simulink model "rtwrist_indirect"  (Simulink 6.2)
settings: Solver=ode45  SolverMode=SingleTasking  StartTime=0.0  StopTime=inf  FixedStep=h  RelTol=1e-3  AbsTol=1e-6
PreLoadFcn:
  | hwinit
StartFcn:
  | hwinit
StopFcn:
  | rtunload
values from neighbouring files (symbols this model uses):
  adingain = [1.2*(pi*2/620/3)*[1 -1 -1 1 1 1] 1]    [hwinit.m]
  adinoffs = [-421 -511 -568 -518 -521 -410    0]    [hwinit.m]
  daoutgain = 127*[1 -1 -1 1 1 1 1]    [hwinit.m]
  daoutoffs = 127*[1 1 1 1 0.98 1 0]    [hwinit.m]
  h = 0.01    [design_pol.m]    (also in design_rot.m; design_wrist.m; rtrobot_init.m = 0.05; simpleregret.m = cfg.h)
  joint = [1 2 3 4 5]    [design_pol.m]    (also in design_rot.m = [1 5]; design_wrist.m = [5]; rtrobot_init.m = joint(:)+(0:6:6*(n-1))')
  Kd = [0.4 0.1 0.1]    [design_pol.m]    (also in design_rot.m = [0.3 0.1]; design_wrist.m = 0.01; mc_approx_vectorized.m = cfg.Kd)
  Ki = [0.6 0.3 0.9]/3    [design_pol.m]    (also in design_rot.m = [0.1 0.1]; design_wrist.m = 0)
  Kp = [0.5 0.2 1.0]    [design_pol.m]    (also in design_rot.m = [0.4 2]; design_wrist.m = 1.5)
undefined symbols (not defined in the file or in its folder): COM1, No
libraries: xpclib x4, rtlib x1, simulink x1

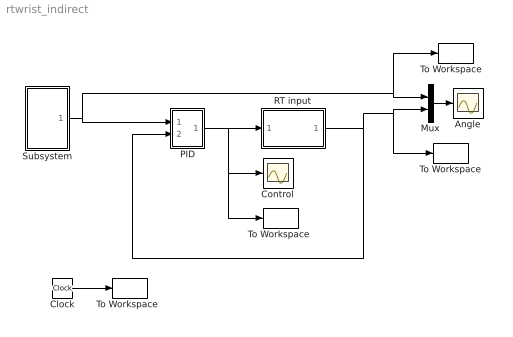
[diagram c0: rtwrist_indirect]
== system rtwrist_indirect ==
  Angle : Scope
  Clock : Clock
  Control : Scope
  Mux : Mux  Inputs=2
  PID : Subsystem
  RT input : Subsystem  InitFcn=rtclear all  mask{h=h, joint=joint, Port=COM1, laser=No, gripper=No}
      mask prompts: h "Sample time [s]:"; joint "Joints to control (e.g., [1 2 4])"; Port "Serial port:"; laser "Enable laser input"; gripper "Enable gripper current sensor"
      mask init:
      | hwinit;
      | sen = joint(:);                             % read joint angles
      | if strcmp(gripper,'Yes'),                   % if gripper current desired
      |     sen = [sen; 7];                         % add to the list
      | end;    
      |                                             
      | n = length(sen);                            % number of sensors to be read
      | sen = sen+(0:7:7*(n-1))';                   % convert into sequential index
      | sen_select = zeros(7,n);                    % prepare zeros
      | sen_select(sen) = 1;                        % assign 1 at the right places
      | 
      | act = joint(:);                             % control joint actuators
      | if strcmp(laser,'Yes'),                     % if laser desired
      |     act = [act; 7];                         % add to the list
      | end;    
      |                                             
      | n = length(act);                            % number of actuators to be controlled
      | act = act+(0:7:7*(n-1))';                   % convert into sequential index
      | act_select = zeros(7,n);                    % prepare zeros
      | act_select(act) = 1;                        % assign 1 at the right places
      | 
      | rtrobot_init(Port);
  Subsystem : Subsystem
  To Workspace : ToWorkspace  VariableName=y  SampleTime=h  SaveFormat=Array
  "To Workspace " : ToWorkspace  VariableName=u  SampleTime=h  SaveFormat=Array
  "To Workspace  " : ToWorkspace  VariableName=t  SampleTime=h  SaveFormat=Array
  "To Workspace   " : ToWorkspace  VariableName=r  SampleTime=h  SaveFormat=Array
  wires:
  Mux/1 -> Angle/1
  Subsystem/1(out_1) -> PID/1(in_1), Mux/1, "To Workspace   "/1
  RT input/1(Angles) -> PID/2(in_2), Mux/2, To Workspace/1
  PID/1(out_1) -> Control/1, "To Workspace "/1, RT input/1(Motors)
  Clock/1 -> "To Workspace  "/1

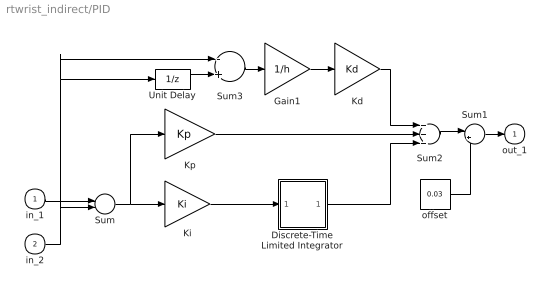
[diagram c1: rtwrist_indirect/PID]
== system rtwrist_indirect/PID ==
  in_1 : Inport  Port=1  LatchInput=off
  in_2 : Inport  Port=2  LatchInput=off
  Discrete-Time Limited Integrator : Subsystem  mask(Discrete-Time Limited Integrator.){}
      mask help: Discrete-Time Limited Integrator.
      mask init:
      | lower_limit=@1;upper_limit=@2;X0=@3;Ts=@4;
  Gain1 : Gain  Gain=1/h  SampleTime=h
  Kd : Gain  Gain=Kd  SampleTime=h
  Ki : Gain  Gain=Ki  SampleTime=h
  Kp : Gain  Gain=Kp  SampleTime=h
  Sum : Sum  Inputs=+-  SampleTime=h
  Sum1 : Sum  Inputs=|++
  Sum2 : Sum  Inputs=+++
  Sum3 : Sum  Inputs=-+  SampleTime=h
  Unit Delay : UnitDelay  SampleTime=h
  offset : Constant  Value=0.03
  out_1 : Outport  InitialOutput=0
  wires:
  Discrete-Time Limited Integrator/1(out_1) -> Sum2/3
  Ki/1 -> Discrete-Time Limited Integrator/1(in_1)
  Sum/1 -> Ki/1, Kp/1
  Gain1/1 -> Kd/1
  Sum3/1 -> Gain1/1
  Kp/1 -> Sum2/2
  Kd/1 -> Sum2/1
  Unit Delay/1 -> Sum3/2
  in_1/1 -> Sum/1
  in_2/1 -> Sum/2, Unit Delay/1, Sum3/1
  Sum2/1 -> Sum1/1
  Sum1/1 -> out_1/1
  offset/1 -> Sum1/2

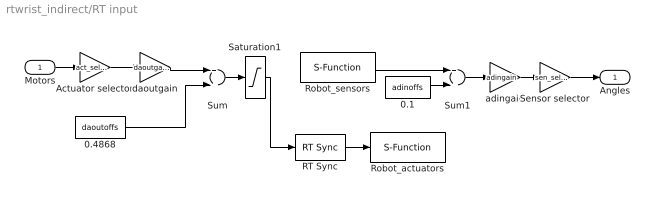
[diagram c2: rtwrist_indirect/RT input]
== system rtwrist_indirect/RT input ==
  Motors : Inport  Port=1  LatchInput=off
  0.1 : Constant  Value=adinoffs
  0.4868 : Constant  Value=daoutoffs
  Actuator selector : Gain  Gain=act_select  Multiplication=Matrix(K*u)
  RT Sync : rtlib/RT Sync
  Robot_actuators : S-Function  FunctionName=sfserialout  Parameters=Ts, com  mask(Serial Out){Ts=h, Port=Port}
      mask prompts: Ts "Sample time:"; Port "Serial port:"
      mask help: Serial line output block
      mask init:
      | com = xserial('Port',Port,'Baudrate',115200);
  Robot_sensors : S-Function  FunctionName=sfserialin  Parameters=Ts, com  mask(Serial Out){Ts=h, Port=Port}
      mask prompts: Ts "Sample time:"; Port "Serial port:"
      mask help: Serial line output block
      mask init:
      | com = xserial('Port',Port,'Baudrate',115200);
  Saturation1 : Saturate  UpperLimit=255  LowerLimit=0
  Sensor selector : Gain  Gain=sen_select'  Multiplication=Matrix(K*u)
  Sum : Sum
  Sum1 : Sum
  adingain : Gain  Gain=adingain
  daoutgain : Gain  Gain=daoutgain
  Angles : Outport
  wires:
  RT Sync/1 -> Robot_actuators/1
  Actuator selector/1 -> daoutgain/1
  Sensor selector/1 -> Angles/1
  Saturation1/1 -> RT Sync/1
  daoutgain/1 -> Sum/1
  adingain/1 -> Sensor selector/1
  Robot_sensors/1 -> Sum1/1
  0.1/1 -> Sum1/2
  Sum1/1 -> adingain/1
  Motors/1 -> Actuator selector/1
  0.4868/1 -> Sum/2
  Sum/1 -> Saturation1/1

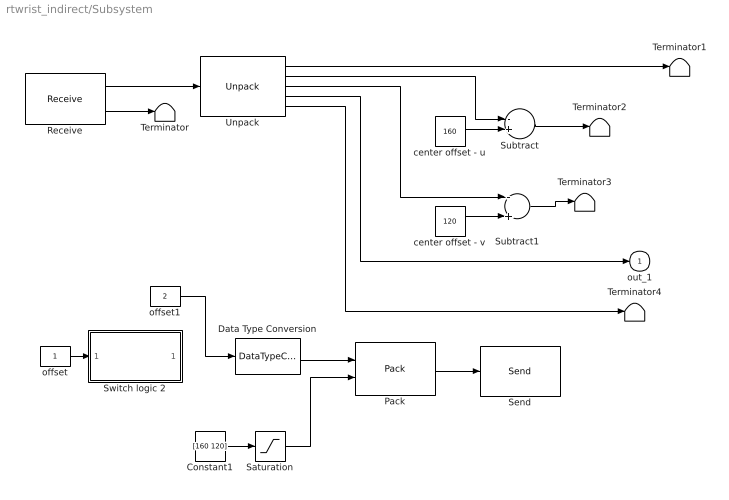
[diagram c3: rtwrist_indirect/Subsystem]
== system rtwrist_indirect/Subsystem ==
  Constant1 : Constant  Value=[160 120]
  Data Type Conversion : DataTypeConversion  OutDataTypeMode=uint8
  Pack : xpclib/UDP/Pack  datatypes={'uint8','double'}  byteAlign=4
  Receive : xpclib/UDP/Receive  ipAddress=127.0.0.1  ipPort=6907  width=40  sampletime=h
  Saturation : Saturate  UpperLimit=[320 240]  LowerLimit=[0 0]
  Send : xpclib/UDP/Send  ipAddress=127.0.0.1  ipPort=6906  localPort=-1  sampletime=h
  Subtract : Sum  Inputs=-+  OutScaling=2^-10
  Subtract1 : Sum  Inputs=-+  OutScaling=2^-10
  Switch logic 2 : Subsystem
  Terminator{,1..4} (5 alike) : Terminator
  Unpack : xpclib/UDP/Unpack  dimensions={1,1,1,1,1}  datatypes={'double','double','double','double','double'}  byteAlign=4
  center offset - u : Constant  Value=160
  center offset - v : Constant  Value=120
  offset : Constant
  offset1 : Constant  Value=2
  out_1 : Outport  InitialOutput=0
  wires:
  Receive/2 -> Terminator/1
  Receive/1 -> Unpack/1
  Unpack/1 -> Terminator1/1
  center offset - u/1 -> Subtract/2
  center offset - v/1 -> Subtract1/2
  Unpack/2 -> Subtract/1
  Unpack/3 -> Subtract1/1
  Unpack/4 -> out_1/1
  Subtract/1 -> Terminator2/1
  Unpack/5 -> Terminator4/1
  Pack/1 -> Send/1
  offset/1 -> Switch logic 2/1(In1)
  Constant1/1 -> Saturation/1
  Data Type Conversion/1 -> Pack/1
  Saturation/1 -> Pack/2
  offset1/1 -> Data Type Conversion/1
  Subtract1/1 -> Terminator3/1

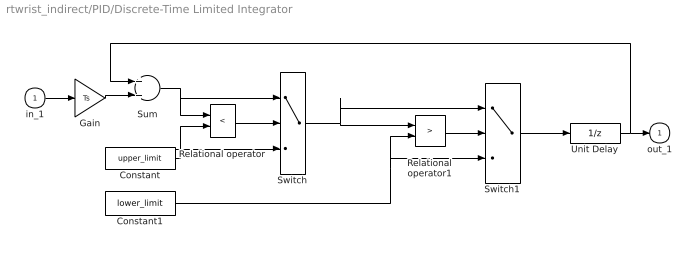
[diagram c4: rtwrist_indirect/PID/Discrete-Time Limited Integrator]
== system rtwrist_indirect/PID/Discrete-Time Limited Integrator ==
  in_1 : Inport  Port=1  LatchInput=off
  Constant : Constant  Value=upper_limit
  Constant1 : Constant  Value=lower_limit
  Gain : Gain  Gain=Ts
  Relational operator : RelationalOperator  Operator=<
  Relational operator1 : RelationalOperator  Operator=>
  Sum : Sum
  Switch : Switch  Threshold=0.5
  Switch1 : Switch  Threshold=0.5
  Unit Delay : UnitDelay  X0=X0  SampleTime=Ts
  out_1 : Outport  InitialOutput=0
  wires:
  in_1/1 -> Gain/1
  Relational operator/1 -> Switch/2
  Sum/1 -> Relational operator/1, Switch/1
  Gain/1 -> Sum/2
  Constant/1 -> Relational operator/2, Switch/3
  Switch/1 -> Switch1/1, Relational operator1/1
  Relational operator1/1 -> Switch1/2
  Constant1/1 -> Switch1/3, Relational operator1/2
  Switch1/1 -> Unit Delay/1
  Unit Delay/1 -> Sum/1, out_1/1

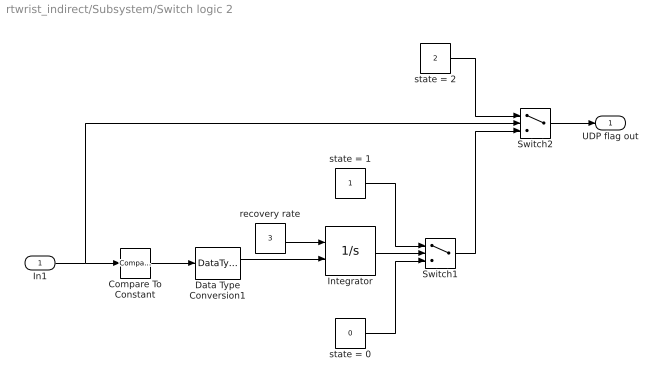
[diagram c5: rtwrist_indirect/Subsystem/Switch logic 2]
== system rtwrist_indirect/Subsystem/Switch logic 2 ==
  In1 : Inport  Port=1  LatchInput=off
  Compare To Constant : simulink/Logic and Bit Operations/Compare To Constant  relop=<  const=1  LogicOutDataTypeMode=uint8  ZeroCross=off
  Data Type Conversion1 : DataTypeConversion  OutDataTypeMode=boolean
  Integrator : Integrator  ExternalReset=rising  LimitOutput=on  UpperSaturationLimit=1  LowerSaturationLimit=0
  Switch1 : Switch  Threshold=0.5
  Switch2 : Switch  Threshold=1
  recovery rate : Constant  Value=3
  state = 0 : Constant  Value=0
  state = 1 : Constant
  state = 2 : Constant  Value=2
  UDP flag out : Outport
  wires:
  state = 1/1 -> Switch1/1
  state = 0/1 -> Switch1/3
  Integrator/1 -> Switch1/2
  Data Type Conversion1/1 -> Integrator/2
  recovery rate/1 -> Integrator/1
  state = 2/1 -> Switch2/1
  Compare To Constant/1 -> Data Type Conversion1/1
  Switch1/1 -> Switch2/3
  Switch2/1 -> UDP flag out/1
  In1/1 -> Compare To Constant/1, Switch2/2
